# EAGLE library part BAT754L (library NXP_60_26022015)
Schottky barrier triple diode Three internal (galvanic) isolated silicon epitaxial Schottky barrier diodes in a SOT363 small SMD plastic package. AAL Eindhoven MK
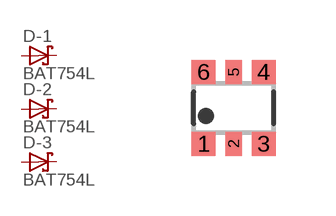
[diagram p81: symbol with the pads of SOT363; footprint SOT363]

Designator prefix D; gates -1=DIODE_SCHOTTKY -2=DIODE_SCHOTTKY -3=DIODE_SCHOTTKY

## BAT754L  [SOT363]
1  -1:A  pas
2  -2:A  pas
3  -3:A  pas
4  -3:K  pas
5  -2:K  pas
6  -1:K  pas

## Footprint SOT363 (pad centres in mm)
SOT363 Plastic surface-mounted package; 6 leads JEDEC: -- IEC: -- JEITA: SC-88
smd 0.6 x 0.6: 1 -0.75,-0.9; 3 0.75,-0.9; 4 0.75,0.9; 6 -0.75,0.9
smd 0.4 x 0.6: 2 0,-0.9; 5 0,0.9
